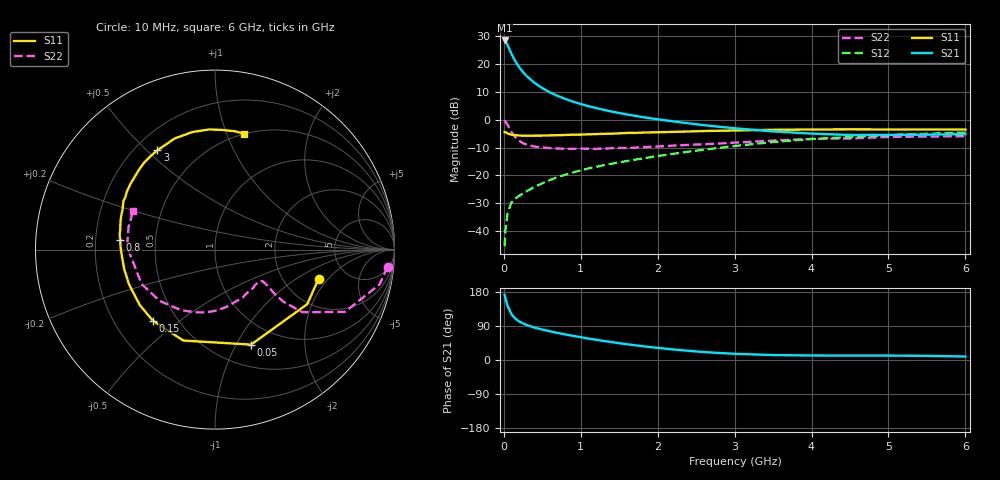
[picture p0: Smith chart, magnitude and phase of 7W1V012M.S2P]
! Infineon Technologies  Discrete & RF Semiconductors
! BFS17W
! Si NPN RF Bipolar Junction Transistor in SOT323
! VCE = 1 V  IC = 12 mA
! Common Emitter S-Parameters:  August  1999
# GHz  S  MA  R  50
!  f  S11  S21  S12  S22
! GHz  MAG  ANG  MAG  ANG  MAG  ANG  MAG  ANG
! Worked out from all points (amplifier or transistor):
!   36 points, 10 MHz to 6 GHz, reference 50 ohm
!   highest |S21| = 28.5 dB at 10 MHz (marker M1)
!   |S21| within 3 dB of that: start of sweep to 70.11 MHz
!   unconditionally stable (mu >= 1): 297.5 MHz to end of sweep
!   at 250 MHz: K = 0.92, MSG = 21.8 dB, |S12| = -26.5 dB
!   at 1.4 GHz: K = 1.31, MAG = 6.0 dB, |S12| = -15.8 dB
!   at 6 GHz: K = 1.12, MAG = -2.4 dB, |S12| = -4.6 dB
!   S11 on the Smith chart (normalised r, x): 10 MHz: 3.13, -1.58; 50 MHz: 0.74, -1.15; 150 MHz: 0.37, -0.40; 800 MHz: 0.31, +0.05; 3 GHz: 0.29, +0.54; 6 GHz: 0.50, +1.16
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0.01  0.5996 -15.6  26.7 171.8  0.0053 83.3  0.9666 -5.7
0.02  0.5972 -30.6  25.96 163.0  0.01 75.1  0.9366 -12.0
0.05  0.5662 -69.2  21.83 141.8  0.0214 63.8  0.803 -25.6
0.1  0.5366 -109.2  15.26 120.8  0.0325 52.3  0.5992 -35.6
0.15  0.526 -131.2  11.21 109.0  0.0381 49.1  0.4808 -37.3
0.2  0.5206 -143.6  8.777 101.7  0.0428 50.8  0.418 -36.7
0.25  0.5146 -152.4  7.159 96.4  0.0473 51.6  0.378 -35.4
0.3  0.5164 -158.4  6.039 92.2  0.0521 53.2  0.356 -34.6
0.4  0.5174 -167.7  4.594 85.5  0.0619 56.3  0.3277 -33.8
0.5  0.5182 -173.6  3.703 80.3  0.0718 58.8  0.3165 -33.7
0.6  0.5222 -178.2  3.099 75.7  0.0821 60.4  0.3086 -34.9
0.7  0.5272 177.7  2.681 71.4  0.093 61.3  0.3034 -36.9
0.8  0.531 174.1  2.363 67.4  0.1021 61.5  0.2993 -39.5
1.1  0.5462 164.7  1.753 56.6  0.1327 62.6  0.3001 -48.3
1.3  0.5574 159.1  1.505 50.1  0.1521 62.3  0.3016 -55.7
1.6  0.5779 151.9  1.243 41.6  0.1806 61.9  0.31 -66.8
2.2  0.6035 138.0  0.934 27.8  0.2435 60.2  0.3413 -89.9
3  0.6397 120.1  0.702 16.4  0.3365 54.6  0.3868 -119.5
3.5  0.6585 110.0  0.616 13.0  0.3967 49.5  0.4207 -137.2
4.5  0.6704 92.7  0.531 11.7  0.4868 36.9  0.459 -169.8
5.5  0.6687 80.4  0.538 10.9  0.5591 25.8  0.498 165.4
6  0.6652 75.7  0.552 9.2  0.5882 20.5  0.5049 154.5
